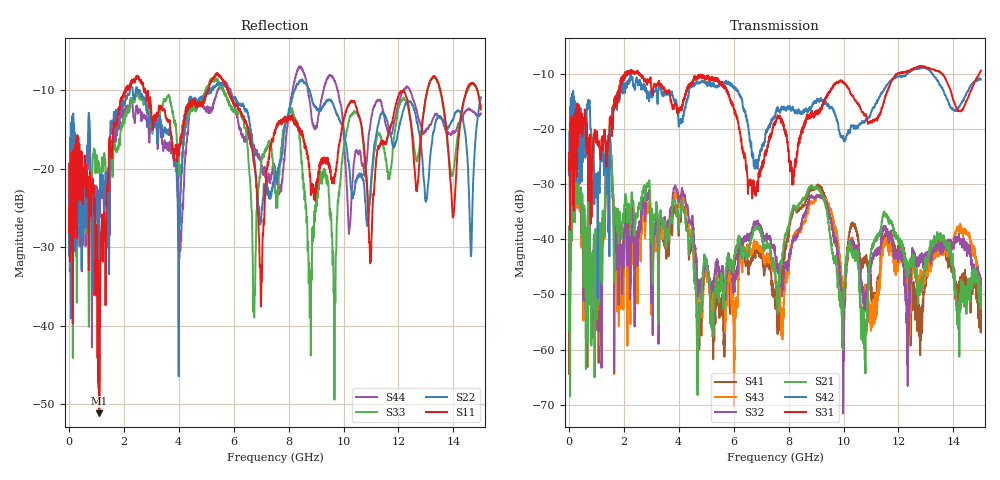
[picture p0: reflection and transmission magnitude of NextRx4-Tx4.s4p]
!  = SDD11
!  = SDD12
!  = SDC11
!  = SDC12
!  = SDD21
!  = SDD22
!  = SDC21
!  = SDC22
!  = SCD11
!  = SCD12
!  = SCC11
!  = SCC12
!  = SCD21
!  = SCD22
!  = SCC21
!  = SCC22
! FILE: N:\QM 2007\Prüfprotokolle\Highspeed\Konfektionierte Ltg\L45593-D106\D30\8216\0002\Next  Platine 1\NextRx4-Tx4.s4p
# MHz S DB R 50.00
! FREQ  S11  S12  S13  S14
!  S21  S22  S23  S24
!  S31  S32  S33  S34
!  S41  S42  S43  S44
!  DB  ANG  DB  ANG  DB  ANG  DB  ANG
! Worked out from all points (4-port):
!   2999 points, 10 MHz to 15 GHz, reference 50 ohm
!   strongest paths, dB at 10 MHz, 3.755 GHz, 7.505 GHz, 11.26 GHz, 15 GHz:
!     S31: -24.6, -15.7, -19.3, -18.0, -9.5
!     S42: -25.2, -13.2, -17.9, -14.9, -11.1
!     S21: -49.2, -36.7, -45.1, -39.2, -49.4
!     S32: -49.7, -34.4, -42.6, -41.5, -47.2
!     S43: -53.4, -36.4, -46.5, -49.9, -50.3
!     S41: -52.9, -39.3, -52.0, -47.7, -52.4
!   lowest |S11| = -51.1 dB at 1.11 GHz (marker M1), VSWR 1.01, Z = 49.9 + j0.26 ohm
!   |S11| at or under -10 dB: start of sweep to 2.068 GHz; 2.781 GHz to 5.055 GHz (2.274 GHz wide, 58 % of centre); 5.79 GHz to 13.05 GHz (7.256 GHz wide, 77 % of centre)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
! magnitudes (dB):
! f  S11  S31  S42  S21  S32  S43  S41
! 10 MHz  -19.4  -24.6  -25.2  -49.2  -49.7  -53.4  -52.9
! 1.11 GHz  -51.1  -23.3  -30.8  -38.4  -42.4  -41.0  -38.5
! 2.48 GHz  -8.2  -10.0  -11.3  -35.7  -41.0  -41.5  -38.6
! 4.71 GHz  -11.9  -10.4  -11.8  -55.3  -49.8  -53.4  -55.3
! 8.785 GHz  -20.7  -17.5  -16.6  -30.7  -32.3  -33.3  -31.3
! 10.77 GHz  -18.3  -17.5  -18.8  -61.7  -52.4  -48.9  -44.0
! 15 GHz  -12.5  -9.5  -11.1  -49.4  -47.2  -50.3  -52.4
